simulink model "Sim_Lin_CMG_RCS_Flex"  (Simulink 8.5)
settings: Solver=ode5  StartTime=0.0  StopTime=3000  FixedStep=Ts/10  RelTol=1e-3
InitFcn:
  | start
StopFcn:
  | Pl
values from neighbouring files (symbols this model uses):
  com_dir = com_dir/sqrt(com_dir'*com_dir)    [start.m]    (also in start1.m; start2.m; start3.m)
  d2r = pi/180    (= 0.0174532925199)    [start.m]    (also in Dead_Band_DF.m; start1.m; start2.m; start3.m)
  J = [0.119416e9, -0.476e7,   -0.1216e7;     -0.476e7,     0.40408e8, -0.30121e6;     -0.1216e7,   -0.30121e6,  0.110166e9]    [start.m]    (also in start1.m; start2.m; start3.m)
  KshC = 2*Wdot_Lim_CMG/WlimC    [start.m]    (also in start1.m; start2.m; start3.m)
  KshR = 2*Wdot_Lim_RCS/WlimR    [start.m]    (also in start1.m; start2.m; start3.m)
  nt = 12    [start.m]    (also in start1.m; start2.m; start3.m)
  omg = 20*wo    (= 0.022)    [start.m]    (also in start1.m; start2.m; start3.m)
  r2d = 180/pi    (= 57.2957795131)    [start.m]    (also in start1.m; start2.m; start3.m)
  Th = 20    [start.m]    (also in start1.m; start2.m; start3.m)
  thecmd = 3    [start.m]    (also in start1.m = 0.1; start2.m = 20; start3.m = 20)
  Wdot_Lim_CMG = 0.0001*d2r    (= 1.74532925199e-06)    [start.m]    (also in start1.m; start2.m; start3.m)
  Wdot_Lim_RCS = 0.02*d2r    (= 0.000349065850399)    [start.m]    (also in start1.m; start2.m; start3.m)
  Wlim_CMG = 0.01*d2r    (= 0.000174532925199)    [start.m]    (also in start1.m; start2.m; start3.m)
  Wlim_RCS = 0.6*d2r    (= 0.010471975512)    [start.m]    (also in start1.m; start2.m; start3.m)
  wo = 0.0011    [start.m]    (also in start1.m; start2.m; start3.m)
  zeb = 0.95    [start.m]    (also in start1.m; start2.m; start3.m)
undefined symbols (not defined in the file or in its folder): Af, Bf, Cf, Df, Phase_Plane, Torq_Lim, Wlim

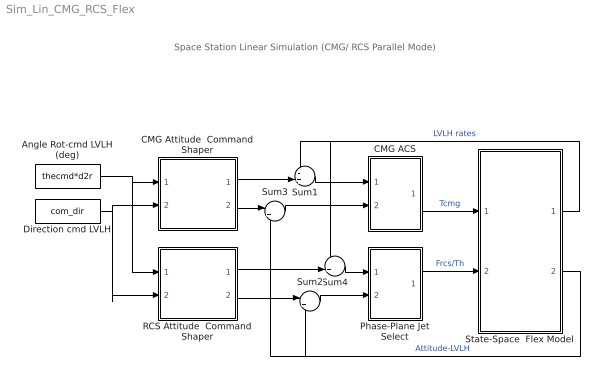
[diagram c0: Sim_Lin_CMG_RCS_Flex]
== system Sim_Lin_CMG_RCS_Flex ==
  note: Space Station Linear Simulation (CMG/ RCS Parallel Mode)
  Angle Rot-cmd LVLH (deg) : Constant  Value=thecmd*d2r
  CMG ACS : Subsystem
  CMG Attitude  Command Shaper : Subsystem
  Direction cmd LVLH : Constant  Value=com_dir
  Phase-Plane Jet Select : Subsystem
  RCS Attitude  Command Shaper : Subsystem
  State-Space  Flex Model : Subsystem
  Sum1 : Sum  Inputs=-+|
  Sum2 : Sum  Inputs=|+-
  Sum3 : Sum  Inputs=|+-
  Sum4 : Sum  Inputs=-+|
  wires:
  State-Space  Flex Model/2(att-lv) -> Sum2/2, Sum3/2  "Attitude-LVLH"
  Sum2/1 -> Phase-Plane Jet Select/2(atter)
  State-Space  Flex Model/1(w-lv) -> Sum1/1, Sum4/1  "LVLH rates"
  Direction cmd LVLH/1 -> CMG Attitude  Command Shaper/2(dir), RCS Attitude  Command Shaper/2(dir)
  Angle Rot-cmd LVLH (deg)/1 -> RCS Attitude  Command Shaper/1(cmd), CMG Attitude  Command Shaper/1(cmd)
  Sum1/1 -> CMG ACS/1(wl)
  CMG Attitude  Command Shaper/1(w-cmd) -> Sum1/2
  CMG Attitude  Command Shaper/2(att-cmd) -> Sum3/1
  Sum3/1 -> CMG ACS/2(ater)
  RCS Attitude  Command Shaper/2(att-cmd) -> Sum2/1
  Phase-Plane Jet Select/1(f(i)) -> State-Space  Flex Model/2(Throtle)  "Frcs/Th"
  Sum4/1 -> Phase-Plane Jet Select/1(rater)
  RCS Attitude  Command Shaper/1(w-cmd) -> Sum4/2
  CMG ACS/1(Tq) -> State-Space  Flex Model/1(Tcmg)  "Tcmg"

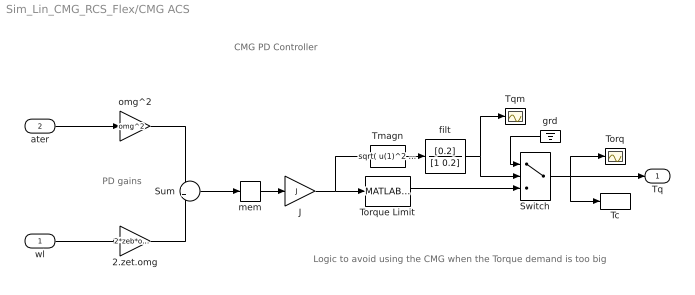
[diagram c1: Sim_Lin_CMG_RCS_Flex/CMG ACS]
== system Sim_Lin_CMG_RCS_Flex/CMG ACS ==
  note: CMG PD Controller
  note: PD gains
  note: Logic to avoid using the CMG when the Torque demand is too big
  wl : Inport
  ater : Inport  Port=2  PortDimensions=3
  2.zet.omg : Gain  Gain=2*zeb*omg
  J : Gain  Gain=J  Multiplication=Matrix(K*u)
  Sum : Sum
  Switch : Switch  Threshold=2500
  Tc : ToWorkspace  VariableName=Tcmg  SampleTime=-1
  Tmagn : Fcn  Expr=sqrt( u(1)^2 + u(2)^2 + u(3)^2 )
  Torq : Scope
  Torque Limit : MATLABFcn  MATLABFcn=Torq_Lim( u(1:3) )  OutputDimensions=3
  Tqm : Scope
  filt : TransferFcn  Numerator=[0.2]  Denominator=[1 0.2]
  grd : Ground
  mem : Memory
  omg^2 : Gain  Gain=omg^2
  Tq : Outport
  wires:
  wl/1 -> 2.zet.omg/1
  Sum/1 -> mem/1
  2.zet.omg/1 -> Sum/2
  ater/1 -> omg^2/1
  omg^2/1 -> Sum/1
  J/1 -> Torque Limit/1, Tmagn/1
  mem/1 -> J/1
  Torque Limit/1 -> Switch/3
  Switch/1 -> Tq/1, Torq/1, Tc/1
  Tmagn/1 -> filt/1
  grd/1 -> Switch/1
  filt/1 -> Switch/2, Tqm/1

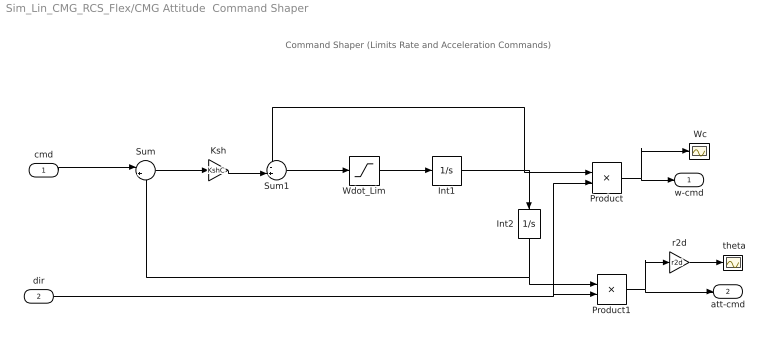
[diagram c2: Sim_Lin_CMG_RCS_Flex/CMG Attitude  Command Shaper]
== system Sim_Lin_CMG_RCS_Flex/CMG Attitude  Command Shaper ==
  note: Command Shaper (Limits Rate and Acceleration Commands)
  cmd : Inport  PortDimensions=1
  dir : Inport  Port=2  PortDimensions=3
  " Wc" : Scope
  " theta" : Scope
  Int1 : Integrator  LimitOutput=on  UpperSaturationLimit=Wlim_CMG  LowerSaturationLimit=-Wlim_CMG
  Int2 : Integrator  UpperSaturationLimit=Wlim  LowerSaturationLimit=-Wlim
  Ksh : Gain  Gain=KshC
  Product : Product
  Product1 : Product
  Sum : Sum  Inputs=|+-
  Sum1 : Sum  Inputs=-+|
  Wdot_Lim : Saturate  UpperLimit=Wdot_Lim_CMG  LowerLimit=-Wdot_Lim_CMG
  r2d : Gain  Gain=r2d
  w-cmd : Outport  PortDimensions=3
  att-cmd : Outport  Port=2  PortDimensions=3
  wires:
  Wdot_Lim/1 -> Int1/1
  Sum1/1 -> Wdot_Lim/1
  Int1/1 -> Product/1, Sum1/1, Int2/1
  Sum/1 -> Ksh/1
  Ksh/1 -> Sum1/2
  Int2/1 -> Sum/2, Product1/1
  cmd/1 -> Sum/1
  dir/1 -> Product/2, Product1/2
  r2d/1 -> " theta"/1
  Product/1 -> w-cmd/1, " Wc"/1
  Product1/1 -> att-cmd/1, r2d/1

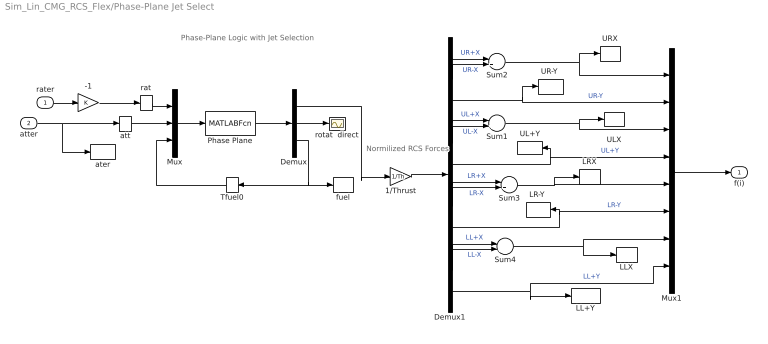
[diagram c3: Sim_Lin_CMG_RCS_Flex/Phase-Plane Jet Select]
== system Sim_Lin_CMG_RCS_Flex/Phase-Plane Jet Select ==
  note: Phase-Plane Logic with Jet Selection
  note: Normilized RCS Forces
  rater : Inport
  atter : Inport  Port=2
  -1 : Gain
  1/Thrust : Gain  Gain=1/Th
  Demux : Demux  Outputs=[nt, 3,1]
  Demux1 : Demux  Outputs=nt
  LL+Y : ToWorkspace  VariableName=LLPY  SampleTime=-1
  LLX : ToWorkspace  VariableName=LLX  SampleTime=-1
  "LR-Y " : ToWorkspace  VariableName=LRNY  SampleTime=-1
  LRX : ToWorkspace  VariableName=LRX  SampleTime=-1
  Mux : Mux  Inputs="[3  3  1]"
  Mux1 : Mux  Inputs=8
  Phase Plane : MATLABFcn  MATLABFcn=Phase_Plane( u(1:3), u(4:6), u(7) )  OutputDimensions=nt + 4
  Sum{1..4} (4 alike) : Sum  Inputs=|+-
  Tfuel0 : Memory
  UL+Y : ToWorkspace  VariableName=ULPY  SampleTime=-1
  ULX : ToWorkspace  VariableName=ULX  SampleTime=-1
  "UR-Y " : ToWorkspace  VariableName=URNY  SampleTime=-1
  URX : ToWorkspace  VariableName=URX  SampleTime=-1
  ater : ToWorkspace  VariableName=atter  SampleTime=-1
  att : Memory
  fuel : ToWorkspace  VariableName=Fuel  SampleTime=-1
  rat : Memory
  rotat  direct : Scope
  f(i) : Outport
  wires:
  Demux/3 -> Tfuel0/1, fuel/1
  att/1 -> Mux/2
  atter/1 -> att/1, ater/1
  rater/1 -> -1/1
  Demux/2 -> rotat  direct/1
  Demux/1 -> 1/Thrust/1
  Tfuel0/1 -> Mux/3
  Phase Plane/1 -> Demux/1
  Mux/1 -> Phase Plane/1
  rat/1 -> Mux/1
  Demux1/1 -> Sum2/1  "UR+X"
  Demux1/2 -> Sum2/2  "UR-X"
  Demux1/4 -> Sum1/1  "UL+X"
  Demux1/5 -> Sum1/2  "UL-X"
  Demux1/7 -> Sum3/1  "LR+X"
  Demux1/8 -> Sum3/2  "LR-X"
  Demux1/10 -> Sum4/1  "LL+X"
  Demux1/11 -> Sum4/2  "LL-X"
  Demux1/3 -> "UR-Y "/1, Mux1/2  "UR-Y"
  -1/1 -> rat/1
  Sum2/1 -> Mux1/1, URX/1
  Sum1/1 -> Mux1/3, ULX/1
  Demux1/6 -> Mux1/4, UL+Y/1  "UL+Y"
  Sum3/1 -> Mux1/5, LRX/1
  Demux1/9 -> Mux1/6, "LR-Y "/1  "LR-Y"
  Sum4/1 -> Mux1/7, LLX/1
  Demux1/12 -> Mux1/8, LL+Y/1  "LL+Y"
  Mux1/1 -> f(i)/1
  1/Thrust/1 -> Demux1/1

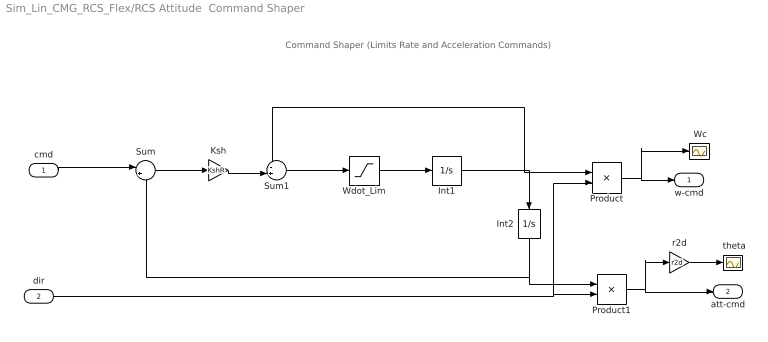
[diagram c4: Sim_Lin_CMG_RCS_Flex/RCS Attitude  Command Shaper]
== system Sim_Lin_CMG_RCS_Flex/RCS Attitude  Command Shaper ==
  note: Command Shaper (Limits Rate and Acceleration Commands)
  cmd : Inport  PortDimensions=1
  dir : Inport  Port=2  PortDimensions=3
  " Wc" : Scope
  " theta" : Scope
  Int1 : Integrator  LimitOutput=on  UpperSaturationLimit=Wlim_RCS  LowerSaturationLimit=-Wlim_RCS
  Int2 : Integrator  UpperSaturationLimit=Wlim  LowerSaturationLimit=-Wlim
  Ksh : Gain  Gain=KshR
  Product : Product
  Product1 : Product
  Sum : Sum  Inputs=|+-
  Sum1 : Sum  Inputs=-+|
  Wdot_Lim : Saturate  UpperLimit=Wdot_Lim_RCS  LowerLimit=-Wdot_Lim_RCS
  r2d : Gain  Gain=r2d
  w-cmd : Outport  PortDimensions=3
  att-cmd : Outport  Port=2  PortDimensions=3
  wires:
  Wdot_Lim/1 -> Int1/1
  Sum1/1 -> Wdot_Lim/1
  Int1/1 -> Product/1, Sum1/1, Int2/1
  Sum/1 -> Ksh/1
  Ksh/1 -> Sum1/2
  Int2/1 -> Sum/2, Product1/1
  cmd/1 -> Sum/1
  dir/1 -> Product/2, Product1/2
  r2d/1 -> " theta"/1
  Product/1 -> w-cmd/1, " Wc"/1
  Product1/1 -> att-cmd/1, r2d/1

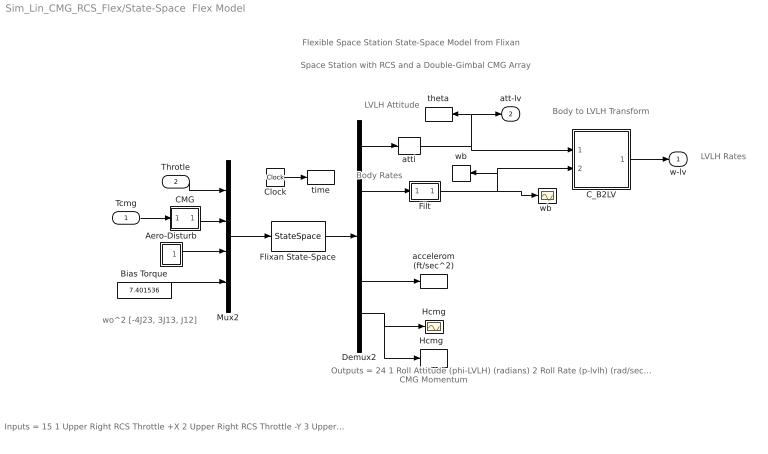
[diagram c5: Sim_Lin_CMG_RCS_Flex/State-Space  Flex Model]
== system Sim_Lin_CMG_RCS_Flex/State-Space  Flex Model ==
  note: Flexible Space Station State-Space Model from Flixan
  note: Space Station with RCS and a Double-Gimbal CMG Array
  note: wo^2 [-4J23, 3J13, J12]
  note: LVLH Attitude
  note: Body Rates
  note: CMG Momentum
  note: Body to LVLH Transform
  note: Outputs = 24 1 Roll Attitude (phi-LVLH) (radians) 2 Roll Rate (p-lvlh) (rad/sec) 3 Pitch Attitude (thet-LVLH) (radians) 4 Pitch Rate (q-lvlh) (rad/sec) 5 Yaw Attitude (psi-LVLH) (radians) 6 Yaw Rate (r-lvlh) (rad/sec) 7 Angle of attack, alfa, (radians) 8 Angle of sideslip, beta, (radian) 9 Change in Altitude, delta-h, (feet) 10 Forward Acceleration (V-dot) (ft/sec) 11 Cross Range Velocity (Vcr) (ft/sec) 12 Rate-Gyro # 1, Roll Rate (Body) (rad/sec) 13 Rate-Gyro # 2, Pitch Rate (Body) (rad/sec) 14 Rate-Gyro # 3, Yaw Rate (Body) (rad/sec) 15 Gyro # 4, Roll Attitude (Body) (radians) 16 Gyro # 5, Pitch Attitude (Body) (radians) 17 Gyro # 6, Yaw Attitude (Body) (radians) 18 Accelerom # 1, (along X), (ft/sec^2) Translat. Accelerat. 19 Accelerom # 2, (along Z), (ft/sec^2) Translat. Accelerat. 20 Accelerom # 3, (along X), (ft/sec^2) Translat. Accelerat. 21 Accelerom # 4, (along Z), (ft/sec^2) Translat. Accelerat. 22 Double Gimbal CMG Momentum Change in X-axis (ft-lb-sec) 23 Double Gimbal CMG Momentum Change in Y-axis (ft-lb-sec) 24 Double Gimbal CMG Momentum Change in Z-axis (ft-lb-sec)
  note: LVLH Rates
  note: Inputs = 15 1 Upper Right RCS Throttle +X 2 Upper Right RCS Throttle -Y 3 Upper Left RCS Throttle +X 4 Upper Left RCS Throttle +Y 5 Lower Right RCS Throttle +X 6 Lower Right RCS Throttle -Y 7 Lower Left RCS Throttle +X 8 Lower Left RCS Throttle +Y 9 Double Gimbal CMG Torque in the X-axis (ft-lb) 10 Double Gimbal CMG Torque in the Y-axis (ft-lb) 11 Double Gimbal CMG Torque in the Z-axis (ft-lb) 12 External Torque Input 1 (ft-lb), direct: 13 External Torque Input 2 (ft-lb), direct: 14 External Torque Input 3 (ft-lb), direct: 15 Ext Torque Direct.=(0.197, -0.5964, -0.7782)
  Tcmg : Inport  PortDimensions=3
  Throtle : Inport  Port=2
  Aero-Disturb : Subsystem
  Bias Torque : Constant  Value=7.401536
  CMG : Subsystem
  C_B2LV : Subsystem
  Clock : Clock
  Demux2 : Demux  Outputs=[11, 3, 3, 4, 3]
  Filt : Subsystem
  Flixan State-Space : StateSpace  A=Af  B=Bf  C=Cf  D=Df  X0=0
  Hcmg : Scope
  "Hcmg  " : ToWorkspace  VariableName=Hcmg  SampleTime=-1
  Mux2 : Mux  Inputs=[8, 3, 3, 1]
  accelerom (ft/sec^2) : ToWorkspace  VariableName=accel  SampleTime=-1
  atti : Selector  InputPortWidth=11  Indices=[1 3 5]
  theta : ToWorkspace  VariableName=theta  SampleTime=-1
  time : ToWorkspace  VariableName=time  SampleTime=-1
  wb : ToWorkspace  VariableName=wb  SampleTime=-1
  "wb " : Scope
  w-lv : Outport
  att-lv : Outport  Port=2
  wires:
  Mux2/1 -> Flixan State-Space/1
  Flixan State-Space/1 -> Demux2/1
  Tcmg/1 -> CMG/1(I)
  Bias Torque/1 -> Mux2/4
  Aero-Disturb/1(Td) -> Mux2/3
  Clock/1 -> time/1
  Throtle/1 -> Mux2/1
  Demux2/5 -> Hcmg/1, "Hcmg  "/1
  Demux2/4 -> accelerom (ft/sec^2)/1
  CMG/1(O) -> Mux2/2
  Demux2/1 -> atti/1
  atti/1 -> att-lv/1, theta/1, C_B2LV/1(atti)
  Demux2/2 -> Filt/1(I)
  C_B2LV/1(wlv) -> w-lv/1
  Filt/1(O) -> "wb "/1, wb/1, C_B2LV/2(wb)

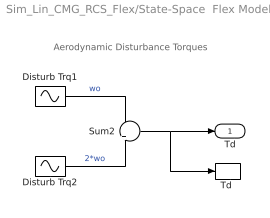
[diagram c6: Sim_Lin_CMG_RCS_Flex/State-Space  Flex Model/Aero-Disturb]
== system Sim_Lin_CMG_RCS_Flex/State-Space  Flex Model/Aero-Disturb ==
  note: Aerodynamic Disturbance Torques
  Disturb Trq1 : Sin  Amplitude=[1, 3, 1]  Bias="[1  8  1]"  Frequency=[wo, wo, wo]  SampleTime=0
  Disturb Trq2 : Sin  Amplitude=[1, 1, 1]*0.5  Frequency=[wo, wo, wo]*2  SampleTime=0
  Sum2 : Sum  Inputs=+|+
  "Td " : ToWorkspace  VariableName=Td  SampleTime=-1
  Td : Outport
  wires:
  Disturb Trq1/1 -> Sum2/1  "wo"
  Sum2/1 -> Td/1, "Td "/1
  Disturb Trq2/1 -> Sum2/2  "2*wo"

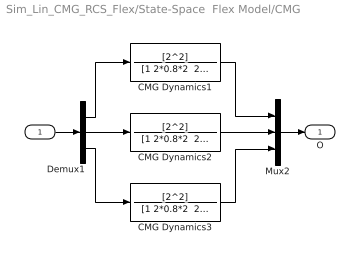
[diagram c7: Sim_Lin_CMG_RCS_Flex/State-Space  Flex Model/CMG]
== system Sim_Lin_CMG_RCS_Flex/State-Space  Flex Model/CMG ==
  I : Inport
  CMG Dynamics1 : TransferFcn  Numerator=[2^2]  Denominator="[1 2*0.8*2  2^2]"
  CMG Dynamics2 : TransferFcn  Numerator=[2^2]  Denominator="[1 2*0.8*2  2^2]"
  CMG Dynamics3 : TransferFcn  Numerator=[2^2]  Denominator="[1 2*0.8*2  2^2]"
  Demux1 : Demux  Outputs=3
  Mux2 : Mux  Inputs=3
  O : Outport
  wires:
  Mux2/1 -> O/1
  I/1 -> Demux1/1
  Demux1/3 -> CMG Dynamics3/1
  Demux1/1 -> CMG Dynamics1/1
  Demux1/2 -> CMG Dynamics2/1
  CMG Dynamics1/1 -> Mux2/1
  CMG Dynamics3/1 -> Mux2/3
  CMG Dynamics2/1 -> Mux2/2

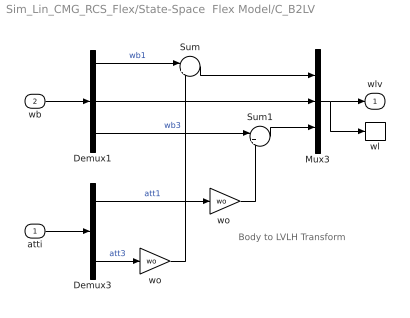
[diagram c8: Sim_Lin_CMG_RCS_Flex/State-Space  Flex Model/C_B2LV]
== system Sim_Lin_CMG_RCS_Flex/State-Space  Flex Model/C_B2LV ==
  note: Body to LVLH Transform
  atti : Inport  PortDimensions=3
  wb : Inport  Port=2  PortDimensions=3
  Demux1 : Demux  Outputs=3
  Demux3 : Demux  Outputs=3
  Mux3 : Mux  Inputs=3
  Sum : Sum  Inputs=|++
  Sum1 : Sum  Inputs=|+-
  wl : ToWorkspace  VariableName=wl  SampleTime=-1
  wo : Gain  Gain=wo
  "wo " : Gain  Gain=wo
  wlv : Outport
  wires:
  "wo "/1 -> Sum1/2
  Demux1/3 -> Sum1/1  "wb3"
  wo/1 -> Sum/2
  Demux1/2 -> Mux3/2
  Demux3/1 -> "wo "/1  "att1"
  Mux3/1 -> wl/1, wlv/1
  wb/1 -> Demux1/1
  atti/1 -> Demux3/1
  Sum1/1 -> Mux3/3
  Demux3/3 -> wo/1  "att3"
  Sum/1 -> Mux3/1
  Demux1/1 -> Sum/1  "wb1"

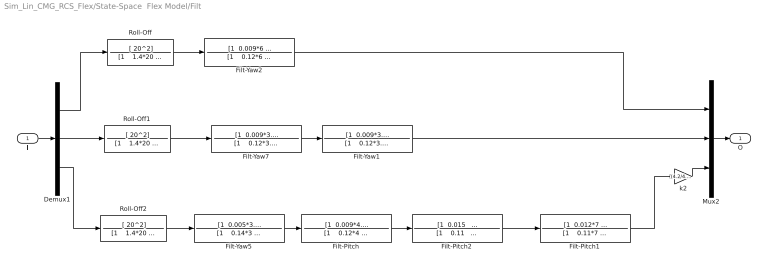
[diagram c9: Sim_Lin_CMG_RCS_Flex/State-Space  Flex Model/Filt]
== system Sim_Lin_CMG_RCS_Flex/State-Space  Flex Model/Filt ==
  I : Inport
  Demux1 : Demux  Outputs=3
  Filt-Pitch : TransferFcn  Numerator="[1  0.009*4.6   4.4^2]"  Denominator="[1    0.12*4    4.2^2]"
  Filt-Pitch1 : TransferFcn  Numerator="[1  0.012*7   6.85^2]"  Denominator="[1    0.11*7    6.85^2]"
  Filt-Pitch2 : TransferFcn  Numerator="[1  0.015   1.14^2]"  Denominator="[1    0.11    1.14^2]"
  Filt-Yaw1 : TransferFcn  Numerator="[1  0.009*3.9   3.93^2]"  Denominator="[1    0.12*3.9    3.93^2]"
  Filt-Yaw2 : TransferFcn  Numerator="[1  0.009*6   5.85^2]"  Denominator="[1    0.12*6    5.85^2]"
  Filt-Yaw5 : TransferFcn  Numerator="[1  0.005*3.1   3.09^2]"  Denominator="[1    0.14*3    3^2]"
  Filt-Yaw7 : TransferFcn  Numerator="[1  0.009*3.5   3.5^2]"  Denominator="[1    0.12*3.5    3.5^2]"
  Mux2 : Mux  Inputs=3
  Roll-Off : TransferFcn  Numerator=[ 20^2]  Denominator="[1    1.4*20    20^2]"
  Roll-Off1 : TransferFcn  Numerator=[ 20^2]  Denominator="[1    1.4*20    20^2]"
  Roll-Off2 : TransferFcn  Numerator=[ 20^2]  Denominator="[1    1.4*20    20^2]"
  k2 : Gain  Gain=(4.2/4.4)*(3/3.09)
  O : Outport
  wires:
  I/1 -> Demux1/1
  Mux2/1 -> O/1
  Demux1/1 -> Roll-Off/1
  Demux1/3 -> Roll-Off2/1
  Demux1/2 -> Roll-Off1/1
  Roll-Off/1 -> Filt-Yaw2/1
  Roll-Off2/1 -> Filt-Yaw5/1
  Roll-Off1/1 -> Filt-Yaw7/1
  Filt-Yaw5/1 -> Filt-Pitch/1
  Filt-Pitch/1 -> Filt-Pitch2/1
  k2/1 -> Mux2/3
  Filt-Yaw7/1 -> Filt-Yaw1/1
  Filt-Yaw1/1 -> Mux2/2
  Filt-Yaw2/1 -> Mux2/1
  Filt-Pitch1/1 -> k2/1
  Filt-Pitch2/1 -> Filt-Pitch1/1
